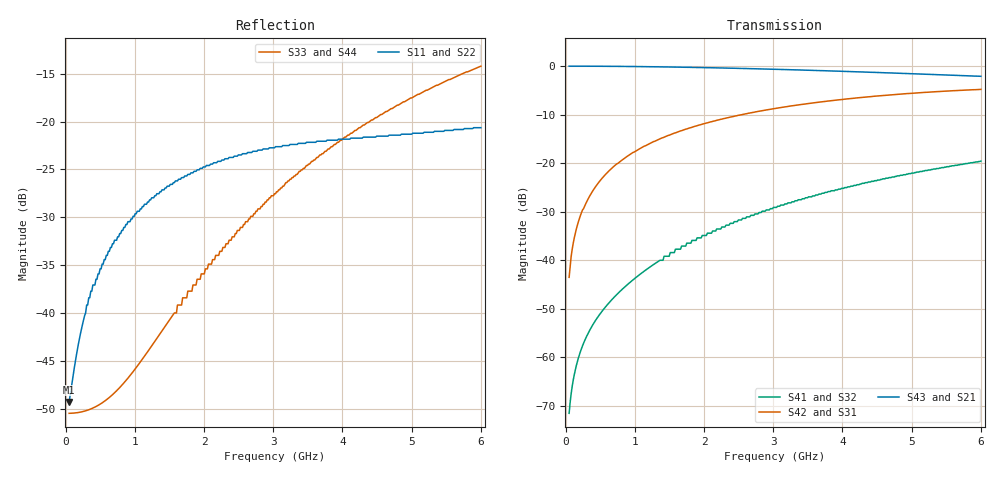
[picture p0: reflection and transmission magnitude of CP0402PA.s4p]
!	AVX THIN FILM OPERATION
!	CP0402 HIGH DIRECTIVITY COUPLERS
!	P/N CP0402PxxxxANTR
!	Network	Analyzer HP8720ES.07.64:Feb23,2000 Serial No.US39172382
!	Hewlett-Packard
!	12 Feb 2007	02:45:57
# MHZ S MA R 50
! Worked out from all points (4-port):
!   400 points, 50 MHz to 6 GHz, reference 50 ohm
!   strongest paths, dB at 50 MHz, 1.541 GHz, 3.032 GHz, 4.524 GHz, 6 GHz:
!     S43: 0.0, -0.2, -0.7, -1.3, -2.1
!     S21: 0.0, -0.2, -0.7, -1.3, -1.9
!     S42: -43.5, -14.0, -8.7, -6.1, -4.8
!     S31: -43.5, -14.0, -8.7, -6.1, -4.8
!     S41: -71.5, -38.4, -29.1, -23.5, -19.6
!     S32: -71.5, -38.4, -29.1, -23.5, -19.6
!   lowest |S11| = -49.3 dB at 50 MHz (marker M1), VSWR 1.01, Z = 50.3 - j0.173 ohm
!   |S11| at or under -10 dB: start of sweep to end of sweep
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50  0.003429 -30.0  0.997 -0.6  0.00667 89.3  0.0002654 -88.8
    0.997 -0.6  0.003429 -30.0  0.0002654 -88.8  0.00667 89.3
    0.00667 89.3  0.0002654 -88.8  0.002988 1.3  0.997 -0.7
    0.0002654 -88.8  0.00667 89.3  0.997 -0.7  0.002988 1.3
94.737  0.004369 -48.1  0.997 -1.2  0.013 88.7  0.0005038 -88.3
        0.997 -1.2  0.004369 -48.1  0.0005038 -88.3  0.013 88.7
        0.013 88.7  0.0005038 -88.3  0.002992 2.4  0.997 -1.4
        0.0005038 -88.3  0.013 88.7  0.997 -1.4  0.002992 2.4
184.211  0.006881 -66.5  0.997 -2.3  0.025 87.5  0.0009864 -87.5
         0.997 -2.3  0.006881 -66.5  0.0009864 -87.5  0.025 87.5
         0.025 87.5  0.0009864 -87.5  0.003017 4.8  0.997 -2.6
         0.0009864 -87.5  0.025 87.5  0.997 -2.6  0.003017 4.8
452.632  0.015 -84.0  0.995 -5.5  0.06 84.0  0.002529 -85.4
         0.995 -5.5  0.015 -84.0  0.002529 -85.4  0.06 84.0
         0.06 84.0  0.002529 -85.4  0.003263 12.8  0.995 -6.5
         0.002529 -85.4  0.06 84.0  0.995 -6.5  0.003263 12.8
1585.965  0.049 -102.9  0.974 -19.1  0.205 69.3  0.013 -90.2
          0.974 -19.1  0.049 -102.9  0.013 -90.2  0.205 69.3
          0.205 69.3  0.013 -90.2  0.01 36.7  0.975 -22.5
          0.013 -90.2  0.205 69.3  0.975 -22.5  0.01 36.7
3375.439  0.077 -113.5  0.909 -39.2  0.399 47.2  0.042 -124.9
          0.909 -39.2  0.077 -113.5  0.042 -124.9  0.399 47.2
          0.399 47.2  0.042 -124.9  0.055 21.0  0.911 -46.8
          0.042 -124.9  0.399 47.2  0.911 -46.8  0.055 21.0
6000  0.093 -104.0  0.802 -64.1  0.575 17.0  0.105 173.9
      0.802 -64.1  0.093 -104.0  0.105 173.9  0.575 17.0
      0.575 17.0  0.105 173.9  0.195 -11.9  0.784 -80.0
      0.105 173.9  0.575 17.0  0.784 -80.0  0.195 -11.9
